| / 7\'7   Xilinx CoolRunner XPLA3 I/O Buffer IBIS File
| \ \   Xilinx Inc.
| / /   2100 Logic Drive
| \_\/.\   San Jose,   CA 95124
[IBIS ver]   2.1
[File name]   xcr3kxl.ibs
[File Rev]   0.4
[Date]   Apr 26, 2002
[Source]   Spice netlist
[Notes]   - Control flag setting:
   SLW=0 - fast slew rate
   SEW=1 - slow slew rate
   - Fix has been made to reduce the non-monotonic
   except the non-monotonic of the pulldown curves
[Disclaimer] The data in this model is derived from SPICE simulations using
   modeling information extracted from the target process. While
   a great deal of care has been take to provide information that
   is accurate, this model is considered preliminary as it has
   not been verified by actual silicon measurement. Treat the
   data in this model as preliminary until actual silicon
   verification is performed.
[Copyright]   Xilinx Inc. All right reserved
|   Component XCR3032XL_PC44[SLW=0]
[Component]   XCR3032XL_PC44[SLW=0]
[Manufacturer]   Xilinx Inc.
[Package]
| variable   typ   min   max
R_pkg   67.500m   66.000m   69.000m
L_pkg   3.950nH   3.600nH   4.300nH
C_pkg   0.900pF   0.800pF   1.000pF
[Pin]  signal_name   model_name   R_pin   L_pin   C_pin
io   PIN   IO_00   NA   NA   NA
| End [Component] XCR3032XL_PC44[SLW=0]
|   Component XCR3032XL_PC44[SLW=1]
[Component]   XCR3032XL_PC44[SLW=1]
[Manufacturer]   Xilinx Inc.
[Package]
| variable   typ   min   max
R_pkg   67.500m   66.000m   69.000m
L_pkg   3.950nH   3.600nH   4.300nH
C_pkg   0.900pF   0.800pF   1.000pF
[Pin]  signal_name   model_name   R_pin   L_pin   C_pin
io   PIN   IO_01   NA   NA   NA
| End [Component] XCR3032XL_PC44[SLW=1]
|   Component XCR3032XL_VQ44[SLW=0]
[Component]   XCR3032XL_VQ44[SLW=0]
[Manufacturer]   Xilinx Inc.
[Package]
| variable   typ   min   max
R_pkg   57.000m   54.000m   60.000m
L_pkg   2.250nH   2.100nH   2.400nH
C_pkg   0.300pF   0.300pF   0.300pF
[Pin]  signal_name   model_name   R_pin   L_pin   C_pin
io   PIN   IO_00   NA   NA   NA
| End [Component] XCR3032XL_VQ44[SLW=0]
|   Component XCR3032XL_VQ44[SLW=1]
[Component]   XCR3032XL_VQ44[SLW=1]
[Manufacturer]   Xilinx Inc.
[Package]
| variable   typ   min   max
R_pkg   57.000m   54.000m   60.000m
L_pkg   2.250nH   2.100nH   2.400nH
C_pkg   0.300pF   0.300pF   0.300pF
[Pin]  signal_name   model_name   R_pin   L_pin   C_pin
io   PIN   IO_01   NA   NA   NA
| End [Component] XCR3032XL_VQ44[SLW=1]
|   Component XCR3032XL_CS48[SLW=0]
[Component]   XCR3032XL_CS48[SLW=0]
[Manufacturer]   Xilinx Inc.
[Package]
| variable   typ   min   max
R_pkg   62.000m   26.000m   98.000m
L_pkg   2.100nH   1.800nH   2.400nH
C_pkg   0.250pF   0.200pF   0.300pF
[Pin]  signal_name   model_name   R_pin   L_pin   C_pin
io   PIN   IO_00   NA   NA   NA
| End [Component] XCR3032XL_CS48[SLW=0]
|   Component XCR3032XL_CS48[SLW=1]
[Component]   XCR3032XL_CS48[SLW=1]
[Manufacturer]   Xilinx Inc.
[Package]
| variable   typ   min   max
R_pkg   62.000m   26.000m   98.000m
L_pkg   2.100nH   1.800nH   2.400nH
C_pkg   0.250pF   0.200pF   0.300pF
[Pin]  signal_name   model_name   R_pin   L_pin   C_pin
io   PIN   IO_01   NA   NA   NA
| End [Component] XCR3032XL_CS48[SLW=1]
|   Component XCR3064XL_CP56[SLW=0]
[Component]   XCR3064XL_CP56[SLW=0]
[Manufacturer]   Xilinx Inc.
[Package]
| variable   typ   min   max
R_pkg   89.000m   75.000m   103.000m
L_pkg   1.850nH   1.500nH   2.200nH
C_pkg   0.350pF   0.300pF   0.400pF
[Pin]  signal_name   model_name   R_pin   L_pin   C_pin
io   PIN   IO_00   NA   NA   NA
| End [Component] XCR3064XL_CP56[SLW=0]
|   Component XCR3064XL_CP56[SLW=1]
[Component]   XCR3064XL_CP56[SLW=1]
[Manufacturer]   Xilinx Inc.
[Package]
| variable   typ   min   max
R_pkg   89.000m   75.000m   103.000m
L_pkg   1.850nH   1.500nH   2.200nH
C_pkg   0.350pF   0.300pF   0.400pF
[Pin]  signal_name   model_name   R_pin   L_pin   C_pin
io   PIN   IO_01   NA   NA   NA
| End [Component] XCR3064XL_CP56[SLW=1]
|   Component XCR3064XL_CS48[SLW=0]
[Component]   XCR3064XL_CS48[SLW=0]
[Manufacturer]   Xilinx Inc.
[Package]
| variable   typ   min   max
R_pkg   112.000m   98.000m   126.000m
L_pkg   2.100nH   1.800nH   2.400nH
C_pkg   0.250pF   0.200pF   0.300pF
[Pin]  signal_name   model_name   R_pin   L_pin   C_pin
io   PIN   IO_00   NA   NA   NA
| End [Component] XCR3064XL_CS48[SLW=0]
|   Component XCR3064XL_CS48[SLW=1]
[Component]   XCR3064XL_CS48[SLW=1]
[Manufacturer]   Xilinx Inc.
[Package]
| variable   typ   min   max
R_pkg   112.000m   98.000m   126.000m
L_pkg   2.100nH   1.800nH   2.400nH
C_pkg   0.250pF   0.200pF   0.300pF
[Pin]  signal_name   model_name   R_pin   L_pin   C_pin
io   PIN   IO_01   NA   NA   NA
| End [Component] XCR3064XL_CS48[SLW=1]
|   Component XCR3064XL_VQ44[SLW=0]
[Component]   XCR3064XL_VQ44[SLW=0]
[Manufacturer]   Xilinx Inc.
[Package]
| variable   typ   min   max
R_pkg   57.000m   54.000m   60.000m
L_pkg   2.250nH   2.100nH   2.400nH
C_pkg   0.300pF   0.300pF   0.300pF
[Pin]  signal_name   model_name   R_pin   L_pin   C_pin
io   PIN   IO_00   NA   NA   NA
| End [Component] XCR3064XL_VQ44[SLW=0]
|   Component XCR3064XL_VQ44[SLW=1]
[Component]   XCR3064XL_VQ44[SLW=1]
[Manufacturer]   Xilinx Inc.
[Package]
| variable   typ   min   max
R_pkg   57.000m   54.000m   60.000m
L_pkg   2.250nH   2.100nH   2.400nH
C_pkg   0.300pF   0.300pF   0.300pF
[Pin]  signal_name   model_name   R_pin   L_pin   C_pin
io   PIN   IO_01   NA   NA   NA
| End [Component] XCR3064XL_VQ44[SLW=1]
|   Component XCR3064XL_VQ100[SLW=0]
[Component]   XCR3064XL_VQ100[SLW=0]
[Manufacturer]   Xilinx Inc.
[Package]
| variable   typ   min   max
R_pkg   101.500m   98.000m   105.000m
L_pkg   5.200nH   4.700nH   5.700nH
C_pkg   0.550pF   0.400pF   0.700pF
[Pin]  signal_name   model_name   R_pin   L_pin   C_pin
io   PIN   IO_00   NA   NA   NA
| End [Component] XCR3064XL_VQ100[SLW=0]
|   Component XCR3064XL_VQ100[SLW=1]
[Component]   XCR3064XL_VQ100[SLW=1]
[Manufacturer]   Xilinx Inc.
[Package]
| variable   typ   min   max
R_pkg   101.500m   98.000m   105.000m
L_pkg   5.200nH   4.700nH   5.700nH
C_pkg   0.550pF   0.400pF   0.700pF
[Pin]  signal_name   model_name   R_pin   L_pin   C_pin
io   PIN   IO_01   NA   NA   NA
| End [Component] XCR3064XL_VQ100[SLW=1]
|   Component XCR3128XL_CS144[SLW=0]
[Component]   XCR3128XL_CS144[SLW=0]
[Manufacturer]   Xilinx Inc.
[Package]
| variable   typ   min   max
R_pkg   109.500m   76.000m   143.000m
L_pkg   2.250nH   1.500nH   3.000nH
C_pkg   0.250pF   0.200pF   0.300pF
[Pin]  signal_name   model_name   R_pin   L_pin   C_pin
io   PIN   IO_00   NA   NA   NA
| End [Component] XCR3128XL_CS144[SLW=0]
|   Component XCR3128XL_CS144[SLW=1]
[Component]   XCR3128XL_CS144[SLW=1]
[Manufacturer]   Xilinx Inc.
[Package]
| variable   typ   min   max
R_pkg   109.500m   76.000m   143.000m
L_pkg   2.250nH   1.500nH   3.000nH
C_pkg   0.250pF   0.200pF   0.300pF
[Pin]  signal_name   model_name   R_pin   L_pin   C_pin
io   PIN   IO_01   NA   NA   NA
| End [Component] XCR3128XL_CS144[SLW=1]
|   Component XCR3128XL_TQ144[SLW=0]
[Component]   XCR3128XL_TQ144[SLW=0]
[Manufacturer]   Xilinx Inc.
[Package]
| variable   typ   min   max
R_pkg   123.500m   117.000m   130.000m
L_pkg   7.950nH   7.100nH   8.800nH
C_pkg   1.000pF   0.800pF   1.200pF
[Pin]  signal_name   model_name   R_pin   L_pin   C_pin
io   PIN   IO_00   NA   NA   NA
| End [Component] XCR3128XL_TQ144[SLW=0]
|   Component XCR3128XL_TQ144[SLW=1]
[Component]   XCR3128XL_TQ144[SLW=1]
[Manufacturer]   Xilinx Inc.
[Package]
| variable   typ   min   max
R_pkg   123.500m   117.000m   130.000m
L_pkg   7.950nH   7.100nH   8.800nH
C_pkg   1.000pF   0.800pF   1.200pF
[Pin]  signal_name   model_name   R_pin   L_pin   C_pin
io   PIN   IO_01   NA   NA   NA
| End [Component] XCR3128XL_TQ144[SLW=1]
|   Component XCR3128XL_VQ100[SLW=0]
[Component]   XCR3128XL_VQ100[SLW=0]
[Manufacturer]   Xilinx Inc.
[Package]
| variable   typ   min   max
R_pkg   101.500m   98.000m   105.000m
L_pkg   5.200nH   4.700nH   5.700nH
C_pkg   0.550pF   0.400pF   0.700pF
[Pin]  signal_name   model_name   R_pin   L_pin   C_pin
io   PIN   IO_00   NA   NA   NA
| End [Component] XCR3128XL_VQ100[SLW=0]
|   Component XCR3128XL_VQ100[SLW=1]
[Component]   XCR3128XL_VQ100[SLW=1]
[Manufacturer]   Xilinx Inc.
[Package]
| variable   typ   min   max
R_pkg   101.500m   98.000m   105.000m
L_pkg   5.200nH   4.700nH   5.700nH
C_pkg   0.550pF   0.400pF   0.700pF
[Pin]  signal_name   model_name   R_pin   L_pin   C_pin
io   PIN   IO_01   NA   NA   NA
| End [Component] XCR3128XL_VQ100[SLW=1]
|   Component XCR3256XL_CS280[SLW=0]
[Component]   XCR3256XL_CS280[SLW=0]
[Manufacturer]   Xilinx Inc.
[Package]
| variable   typ   min   max
R_pkg   259.500m   148.000m   371.000m
L_pkg   5.800nH   2.700nH   8.900nH
C_pkg   0.500pF   0.200pF   0.800pF
[Pin]  signal_name   model_name   R_pin   L_pin   C_pin
io   PIN   IO_00   NA   NA   NA
| End [Component] XCR3256XL_CS280[SLW=0]
|   Component XCR3256XL_CS280[SLW=1]
[Component]   XCR3256XL_CS280[SLW=1]
[Manufacturer]   Xilinx Inc.
[Package]
| variable   typ   min   max
R_pkg   259.500m   148.000m   371.000m
L_pkg   5.800nH   2.700nH   8.900nH
C_pkg   0.500pF   0.200pF   0.800pF
[Pin]  signal_name   model_name   R_pin   L_pin   C_pin
io   PIN   IO_01   NA   NA   NA
| End [Component] XCR3256XL_CS280[SLW=1]
|   Component XCR3256XL_PQ208[SLW=0]
[Component]   XCR3256XL_PQ208[SLW=0]
[Manufacturer]   Xilinx Inc.
[Package]
| variable   typ   min   max
R_pkg   195.500m   195.000m   196.000m
L_pkg   14.200nH   12.500nH   15.900nH
C_pkg   1.800pF   1.600pF   2.000pF
[Pin]  signal_name   model_name   R_pin   L_pin   C_pin
io   PIN   IO_00   NA   NA   NA
| End [Component] XCR3256XL_PQ208[SLW=0]
|   Component XCR3256XL_PQ208[SLW=1]
[Component]   XCR3256XL_PQ208[SLW=1]
[Manufacturer]   Xilinx Inc.
[Package]
| variable   typ   min   max
R_pkg   195.500m   195.000m   196.000m
L_pkg   14.200nH   12.500nH   15.900nH
C_pkg   1.800pF   1.600pF   2.000pF
[Pin]  signal_name   model_name   R_pin   L_pin   C_pin
io   PIN   IO_01   NA   NA   NA
| End [Component] XCR3256XL_PQ208[SLW=1]
|   Component XCR3256XL_TQ144[SLW=0]
[Component]   XCR3256XL_TQ144[SLW=0]
[Manufacturer]   Xilinx Inc.
[Package]
| variable   typ   min   max
R_pkg   123.500m   117.000m   130.000m
L_pkg   7.950nH   7.100nH   8.800nH
C_pkg   1.000pF   0.800pF   1.200pF
[Pin]  signal_name   model_name   R_pin   L_pin   C_pin
io   PIN   IO_00   NA   NA   NA
| End [Component] XCR3256XL_TQ144[SLW=0]
|   Component XCR3256XL_TQ144[SLW=1]
[Component]   XCR3256XL_TQ144[SLW=1]
[Manufacturer]   Xilinx Inc.
[Package]
| variable   typ   min   max
R_pkg   123.500m   117.000m   130.000m
L_pkg   7.950nH   7.100nH   8.800nH
C_pkg   1.000pF   0.800pF   1.200pF
[Pin]  signal_name   model_name   R_pin   L_pin   C_pin
io   PIN   IO_01   NA   NA   NA
| End [Component] XCR3256XL_TQ144[SLW=1]
|   Component XCR3384XL_PQ208[SLW=0]
[Component]   XCR3384XL_PQ208[SLW=0]
[Manufacturer]   Xilinx Inc.
[Package]
| variable   typ   min   max
R_pkg   187.500m   180.000m   195.000m
L_pkg   12.100nH   11.700nH   12.500nH
C_pkg   1.4500pF   1.3000pF   1.6000pF
[Pin]  signal_name   model_name   R_pin   L_pin   C_pin
io   PIN   IO_00   NA   NA   NA
| End [Component] XCR3384XL_PQ208[SLW=0]
|   Component XCR3384XL_PQ208[SLW=1]
[Component]   XCR3384XL_PQ208[SLW=1]
[Manufacturer]   Xilinx Inc.
[Package]
| variable   typ   min   max
R_pkg   187.500m   180.000m   195.000m
L_pkg   12.100nH   11.700nH   12.500nH
C_pkg   1.4500pF   1.3000pF   1.6000pF
[Pin]  signal_name   model_name   R_pin   L_pin   C_pin
io   PIN   IO_01   NA   NA   NA
| End [Component] XCR3384XL_PQ208[SLW=1]
|   Component XCR3384XL_FT256[SLW=0]
[Component]   XCR3384XL_FT256[SLW=0]
[Manufacturer]   Xilinx Inc.
[Package]
| variable   typ   min   max
R_pkg   266.95m   201.300m   332.600m
L_pkg   6.550nH   3.200nH   9.900nH
C_pkg   0.9500pF   0.6000pF   1.3000pF
[Pin]  signal_name   model_name   R_pin   L_pin   C_pin
io   PIN   IO_00   NA   NA   NA
| End [Component] XCR3384XL_FT256[SLW=0]
|   Component XCR3384XL_FT256[SLW=1]
[Component]   XCR3384XL_FT256[SLW=1]
[Manufacturer]   Xilinx Inc.
[Package]
| variable   typ   min   max
R_pkg   266.95m   201.300m   332.600m
L_pkg   6.550nH   3.200nH   9.900nH
C_pkg   0.9500pF   0.6000pF   1.3000pF
[Pin]  signal_name   model_name   R_pin   L_pin   C_pin
io   PIN   IO_01   NA   NA   NA
| End [Component] XCR3384XL_FT256[SLW=1]
| Models and submodels in the file (2): IO_00 (I/O), IO_01 (I/O)
